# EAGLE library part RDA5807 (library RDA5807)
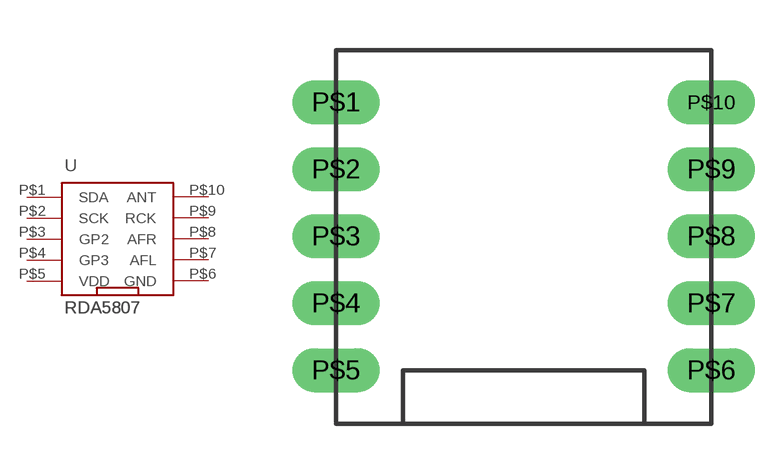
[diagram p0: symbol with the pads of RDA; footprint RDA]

Designator prefix -

## RDA5807  [RDA]
P$1  SDA
P$2  SCK
P$3  GP2
P$4  GP3
P$5  VDD
P$6  GND
P$7  AFL  out
P$8  AFR  out
P$9  RCK  nc
P$10  ANT  in

## Footprint RDA (pad centres in mm)
drill 0.8 pad 1.265 long: P$1 0,8; P$2 0,6; P$3 0,4; P$4 0,2; P$5 0,0; P$6 11.2,0; P$7 11.2,2; P$8 11.2,4; P$9 11.2,6; P$10 11.2,8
